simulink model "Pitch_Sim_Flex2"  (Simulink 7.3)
settings: Solver=ode113  StartTime=0.0  StopTime=100  MaxStep=0.002  RelTol=1e-3
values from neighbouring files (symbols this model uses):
  Aac = [    [actuator_srb.m]    (also in actuator_ssme.m; actuators_5s.m; actuators_5z.m)
  Bac = [    [actuator_srb.m]    (also in actuator_ssme.m; actuators_5s.m; actuators_5z.m)
  Cac = [    [actuator_srb.m]    (also in actuator_ssme.m; actuators_5s.m; actuators_5z.m)
  d2r = 1/r2d    (= 0.0174532925199)    [run.m]
  Dac = [    [actuator_srb.m]    (also in actuator_ssme.m; actuators_5s.m; actuators_5z.m)
undefined symbols (not defined in the file or in its folder): Apf, Asb, Bpf, Bsb, Cpf, Csb, Dpf, Dsb

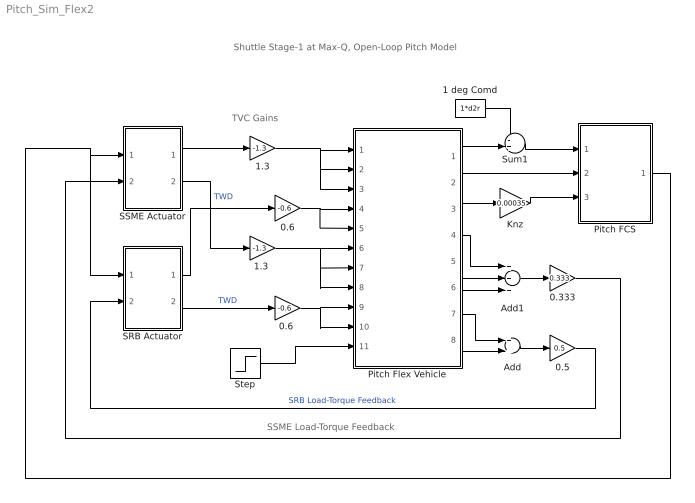
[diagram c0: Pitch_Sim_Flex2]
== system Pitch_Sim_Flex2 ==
  note: SSME Load-Torque Feedback
  note: TVC Gains
  note: Shuttle Stage-1 at Max-Q, Open-Loop Pitch Model
  0.333 : Gain  Gain=0.333  ParameterDataType=sfix(16)  ParameterScaling=2^0  OutDataType=sfix(16)  OutScaling=2^0
  0.5 : Gain  Gain=0.5  ParameterDataType=sfix(16)  ParameterScaling=2^0  OutDataType=sfix(16)  OutScaling=2^0
  0.6 : Gain  Gain=-0.6  ParameterDataType=sfix(16)  ParameterScaling=2^0  OutDataType=sfix(16)  OutScaling=2^0
  "0.6 " : Gain  Gain=-0.6  ParameterDataType=sfix(16)  ParameterScaling=2^0  OutDataType=sfix(16)  OutScaling=2^0
  1 deg Comd : Constant  Value=1*d2r  OutDataType=sfix(16)  OutScaling=2^0  SampleTime=-1
  1.3 : Gain  Gain=-1.3  ParameterDataType=sfix(16)  ParameterScaling=2^0  OutDataType=sfix(16)  OutScaling=2^0
  "1.3 " : Gain  Gain=-1.3  ParameterDataType=sfix(16)  ParameterScaling=2^0  OutDataType=sfix(16)  OutScaling=2^0
  Add : Sum  OutDataType=sfix(16)  OutScaling=2^-10
  Add1 : Sum  Inputs=+++  OutDataType=sfix(16)  OutScaling=2^-10
  Knz : Gain  Gain=0.00035  ParameterDataType=sfix(16)  ParameterScaling=2^0  OutDataType=sfix(16)  OutScaling=2^0
  Pitch FCS : Subsystem
  Pitch Flex Vehicle : Subsystem
  SRB Actuator : Subsystem
  SSME Actuator : Subsystem
  Step : Step  Time=0.5  After=00  SampleTime=0
  Sum1 : Sum  Inputs=-+|  OutDataType=sfix(16)  OutScaling=2^0
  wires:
  SSME Actuator/1(dy) -> 1.3/1
  Pitch FCS/1(DQ_TVC) -> SSME Actuator/1(dy-com), SRB Actuator/1(dy-com)
  1.3/1 -> Pitch Flex Vehicle/1(dy1), Pitch Flex Vehicle/2(dy2), Pitch Flex Vehicle/3(dy3)
  0.6/1 -> Pitch Flex Vehicle/4(dy4), Pitch Flex Vehicle/5(dy5)
  SSME Actuator/2(dy-dd) -> "1.3 "/1  "TWD"
  "1.3 "/1 -> Pitch Flex Vehicle/6(dydd1), Pitch Flex Vehicle/7(dydd2), Pitch Flex Vehicle/8(dydd3)
  "0.6 "/1 -> Pitch Flex Vehicle/9(dydd4), Pitch Flex Vehicle/10(dydd5)
  Pitch Flex Vehicle/3(Nz) -> Knz/1
  SRB Actuator/1(dy) -> 0.6/1
  SRB Actuator/2(dy-dd) -> "0.6 "/1  "TWD"
  Pitch Flex Vehicle/7(TLy4) -> Add/1
  Pitch Flex Vehicle/8(TLy5) -> Add/2
  Add/1 -> 0.5/1
  0.5/1 -> SRB Actuator/2(TL)  "SRB Load-Torque Feedback"
  Add1/1 -> 0.333/1
  Pitch Flex Vehicle/6(TLy3) -> Add1/3
  Pitch Flex Vehicle/5(TLy2) -> Add1/2
  Pitch Flex Vehicle/4(TLy1) -> Add1/1
  0.333/1 -> SSME Actuator/2(TL)
  Pitch Flex Vehicle/2(q-flx) -> Pitch FCS/2(q)
  Pitch Flex Vehicle/1(theta) -> Sum1/2
  Sum1/1 -> Pitch FCS/1(theta)
  1 deg Comd/1 -> Sum1/1
  Step/1 -> Pitch Flex Vehicle/11(WG)
  Knz/1 -> Pitch FCS/3(Nz)

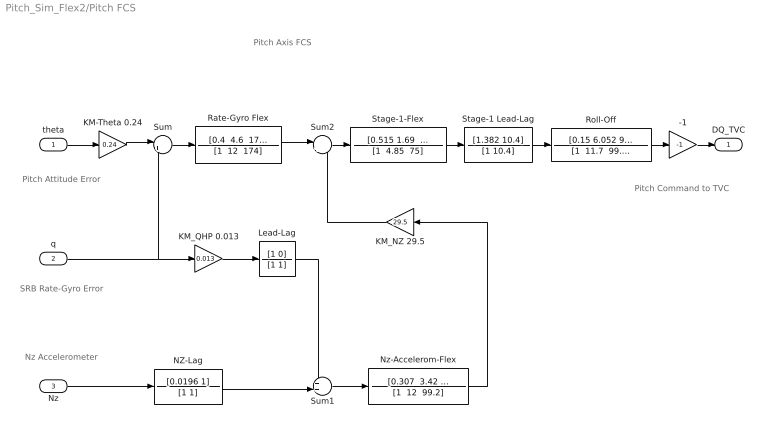
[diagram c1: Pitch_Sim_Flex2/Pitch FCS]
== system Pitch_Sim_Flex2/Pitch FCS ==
  note: Pitch Axis FCS
  note: Nz Accelerometer
  note: Pitch Attitude Error
  note: SRB Rate-Gyro Error
  note: Pitch Command to TVC
  theta : Inport  OutDataType=fixdt(1, 16)  OutScaling=2^0
  q : Inport  Port=2  OutDataType=fixdt(1, 16)  OutScaling=2^0
  Nz : Inport  Port=3  OutDataType=fixdt(1, 16)  OutScaling=2^0
  -1 : Gain  Gain=-1  ParameterDataType=fixdt(1, 16)  ParameterScaling=2^0  OutDataType=fixdt(1, 16)  OutScaling=2^0
  KM-Theta 0.24 : Gain  Gain=0.24  ParameterDataType=fixdt(1, 16)  ParameterScaling=2^0  OutDataType=fixdt(1, 16)  OutScaling=2^0
  KM_NZ 29.5 : Gain  Gain=29.5  ParameterDataType=fixdt(1, 16)  ParameterScaling=2^0  OutDataType=fixdt(1, 16)  OutScaling=2^0
  KM_QHP 0.013 : Gain  Gain=0.013  ParameterDataType=fixdt(1, 16)  ParameterScaling=2^0  OutDataType=fixdt(1, 16)  OutScaling=2^0
  Lead-Lag : TransferFcn  Numerator=[1 0]  Denominator=[1 1]
  NZ-Lag : TransferFcn  Numerator=[0.0196 1]  Denominator=[1 1]
  Nz-Accelerom-Flex : TransferFcn  Numerator="[0.307  3.42  99.2]"  Denominator="[1  12  99.2]"
  Rate-Gyro Flex : TransferFcn  Numerator="[0.4  4.6  174]"  Denominator="[1  12  174]"
  Roll-Off : TransferFcn  Numerator=[0.15 6.052 99.2]  Denominator="[1  11.7  99.2]"
  Stage-1 Lead-Lag : TransferFcn  Numerator=[1.382 10.4]  Denominator=[1 10.4]
  Stage-1-Flex : TransferFcn  Numerator="[0.515 1.69  75]"  Denominator="[1  4.85  75]"
  Sum : Sum  Inputs=|++  OutDataType=fixdt(1, 16)  OutScaling=2^0
  Sum1 : Sum  Inputs=++|  OutDataType=fixdt(1, 16)  OutScaling=2^0
  Sum2 : Sum  Inputs=|++  OutDataType=fixdt(1, 16)  OutScaling=2^0
  DQ_TVC : Outport  OutDataType=fixdt(1, 16)  OutScaling=2^0
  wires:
  theta/1 -> KM-Theta 0.24/1
  KM-Theta 0.24/1 -> Sum/1
  Sum/1 -> Rate-Gyro Flex/1
  q/1 -> Sum/2, KM_QHP 0.013/1
  KM_QHP 0.013/1 -> Lead-Lag/1
  Nz/1 -> NZ-Lag/1
  Stage-1 Lead-Lag/1 -> Roll-Off/1
  Stage-1-Flex/1 -> Stage-1 Lead-Lag/1
  NZ-Lag/1 -> Sum1/2
  Sum1/1 -> Nz-Accelerom-Flex/1
  Lead-Lag/1 -> Sum1/1
  Rate-Gyro Flex/1 -> Sum2/1
  Sum2/1 -> Stage-1-Flex/1
  Nz-Accelerom-Flex/1 -> KM_NZ 29.5/1
  KM_NZ 29.5/1 -> Sum2/2
  Roll-Off/1 -> -1/1
  -1/1 -> DQ_TVC/1

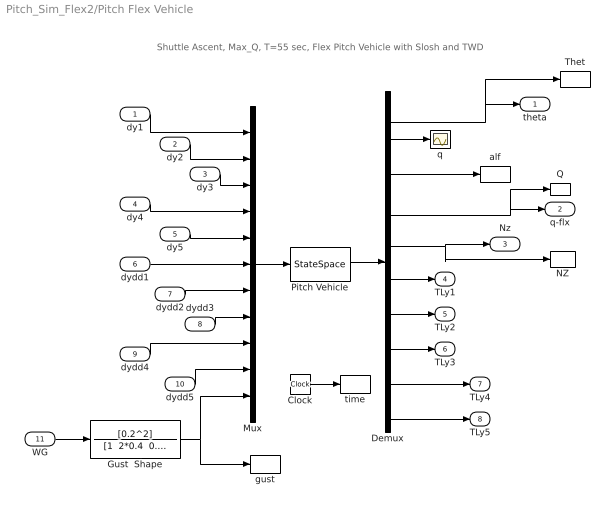
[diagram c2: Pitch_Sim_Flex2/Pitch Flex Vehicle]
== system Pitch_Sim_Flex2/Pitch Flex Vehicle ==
  note: Shuttle Ascent, Max_Q, T=55 sec, Flex Pitch Vehicle with Slosh and TWD
  dy1 : Inport  OutDataType=sfix(16)  OutScaling=2^0
  dy2 : Inport  Port=2  OutDataType=sfix(16)  OutScaling=2^0
  dy3 : Inport  Port=3  OutDataType=sfix(16)  OutScaling=2^0
  dy4 : Inport  Port=4  OutDataType=sfix(16)  OutScaling=2^0
  dy5 : Inport  Port=5  OutDataType=sfix(16)  OutScaling=2^0
  dydd1 : Inport  Port=6  OutDataType=sfix(16)  OutScaling=2^0
  dydd2 : Inport  Port=7  OutDataType=sfix(16)  OutScaling=2^0
  dydd3 : Inport  Port=8  OutDataType=sfix(16)  OutScaling=2^0
  dydd4 : Inport  Port=9  OutDataType=sfix(16)  OutScaling=2^0
  dydd5 : Inport  Port=10  OutDataType=sfix(16)  OutScaling=2^0
  WG : Inport  Port=11  OutDataType=sfix(16)  OutScaling=2^0
  Clock : Clock
  Demux : Demux  Outputs=10
  Gust  Shape : TransferFcn  Numerator=[0.2^2]  Denominator="[1  2*0.4  0.2^2]"
  Mux : Mux  Inputs=11
  NZ : ToWorkspace  VariableName=Nz  SampleTime=-1  SaveFormat=Array
  Pitch Vehicle : StateSpace  A=Apf  B=Bpf  C=Cpf  D=Dpf
  Q : ToWorkspace  VariableName=q  SampleTime=-1  SaveFormat=Array
  Thet : ToWorkspace  VariableName=theta  SampleTime=-1  SaveFormat=Array
  alf : ToWorkspace  VariableName=alpha  SampleTime=-1  SaveFormat=Array
  gust : ToWorkspace  VariableName=Gust  SampleTime=-1  SaveFormat=Array
  q : Scope
  time : ToWorkspace  VariableName=time  SampleTime=-1  SaveFormat=Array
  theta : Outport  OutDataType=sfix(16)  OutScaling=2^0
  q-flx : Outport  Port=2  OutDataType=sfix(16)  OutScaling=2^0
  Nz : Outport  Port=3  OutDataType=sfix(16)  OutScaling=2^0
  TLy1 : Outport  Port=4  OutDataType=sfix(16)  OutScaling=2^0
  TLy2 : Outport  Port=5  OutDataType=sfix(16)  OutScaling=2^0
  TLy3 : Outport  Port=6  OutDataType=sfix(16)  OutScaling=2^0
  TLy4 : Outport  Port=7  OutDataType=sfix(16)  OutScaling=2^0
  TLy5 : Outport  Port=8  OutDataType=sfix(16)  OutScaling=2^0
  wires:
  Pitch Vehicle/1 -> Demux/1
  Mux/1 -> Pitch Vehicle/1
  Demux/2 -> q/1
  Demux/3 -> alf/1
  dy1/1 -> Mux/1
  dy2/1 -> Mux/2
  dy3/1 -> Mux/3
  dy4/1 -> Mux/4
  dy5/1 -> Mux/5
  dydd1/1 -> Mux/6
  dydd2/1 -> Mux/7
  dydd3/1 -> Mux/8
  dydd4/1 -> Mux/9
  dydd5/1 -> Mux/10
  WG/1 -> Gust  Shape/1
  Demux/1 -> theta/1, Thet/1
  Demux/5 -> Nz/1, NZ/1
  Demux/6 -> TLy1/1
  Demux/7 -> TLy2/1
  Demux/8 -> TLy3/1
  Demux/9 -> TLy4/1
  Demux/10 -> TLy5/1
  Demux/4 -> q-flx/1, Q/1
  Gust  Shape/1 -> Mux/11, gust/1
  Clock/1 -> time/1

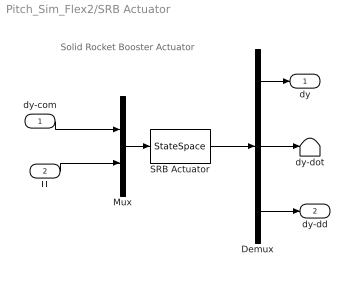
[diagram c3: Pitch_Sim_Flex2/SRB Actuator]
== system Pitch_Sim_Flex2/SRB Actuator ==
  note: Solid Rocket Booster Actuator
  dy-com : Inport  PortDimensions=1  OutDataType=sfix(16)  OutScaling=2^0
  TL : Inport  Port=2  OutDataType=sfix(16)  OutScaling=2^0
  Demux : Demux  Outputs=3
  Mux : Mux  Inputs=2
  SRB Actuator : StateSpace  A=Asb  B=Bsb  C=Csb  D=Dsb
  dy-dot : Terminator
  dy : Outport  OutDataType=sfix(16)  OutScaling=2^0
  dy-dd : Outport  Port=2  OutDataType=sfix(16)  OutScaling=2^0
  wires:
  SRB Actuator/1 -> Demux/1
  Mux/1 -> SRB Actuator/1
  Demux/1 -> dy/1
  dy-com/1 -> Mux/1
  TL/1 -> Mux/2
  Demux/2 -> dy-dot/1
  Demux/3 -> dy-dd/1

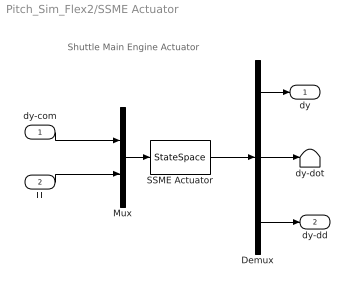
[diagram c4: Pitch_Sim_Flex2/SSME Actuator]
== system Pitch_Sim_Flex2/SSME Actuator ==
  note: Shuttle Main Engine Actuator
  dy-com : Inport  PortDimensions=1  OutDataType=sfix(16)  OutScaling=2^0
  TL : Inport  Port=2  OutDataType=sfix(16)  OutScaling=2^0
  Demux : Demux  Outputs=3
  Mux : Mux  Inputs=2
  SSME Actuator : StateSpace  A=Aac  B=Bac  C=Cac  D=Dac
  dy-dot : Terminator
  dy : Outport  OutDataType=sfix(16)  OutScaling=2^0
  dy-dd : Outport  Port=2  OutDataType=sfix(16)  OutScaling=2^0
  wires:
  SSME Actuator/1 -> Demux/1
  Mux/1 -> SSME Actuator/1
  Demux/1 -> dy/1
  dy-com/1 -> Mux/1
  TL/1 -> Mux/2
  Demux/2 -> dy-dot/1
  Demux/3 -> dy-dd/1
